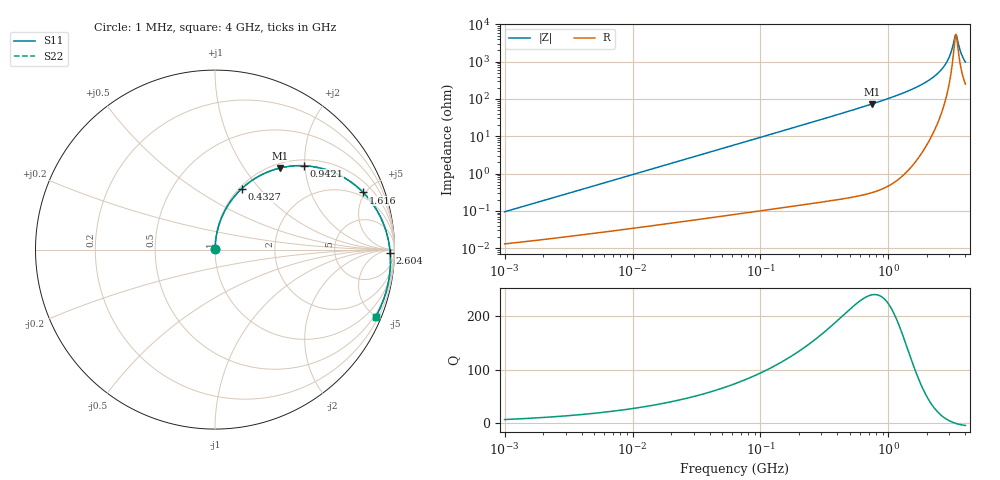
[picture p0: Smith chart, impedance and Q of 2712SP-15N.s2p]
# MHz  S  MA  R  50
!Freq  MagS11  AngS11  MagS21  AngS21  MagS12  AngS12  MagS22  AngS22
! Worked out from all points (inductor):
!   801 points, 1 MHz to 4 GHz, reference 50 ohm
!   read as one part in series: L = 14.9 nH near 1.042 MHz
!   highest Q = 239 at 749.9 MHz (marker M1), where L = 15.7 nH
!   self-resonance near 3.341 GHz
!   S11 on the Smith chart (normalised r, x): 1 MHz: 1.00, +0.00; 432.7 MHz: 1.03, +0.81; 942.1 MHz: 1.13, +1.97; 1.616 GHz: 1.65, +4.84; 2.604 GHz: 48, -41; 4 GHz: 0.38, -4.92
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1  0.0009136 81.8  0.9999 -0.1  0.9999 -0.1  0.0009136 81.8
4.016383  0.003639 86.2  0.9998 -0.2  0.9998 -0.2  0.003639 86.2
15.96482  0.01444 87.4  0.9995 -0.9  0.9995 -0.9  0.01444 87.4
63.45894  0.05729 85.7  0.9976 -3.5  0.9976 -3.5  0.05728 85.7
133.9496  0.1204 82.0  0.9916 -7.4  0.9916 -7.4  0.1203 82.0
252.2445  0.2234 75.8  0.9732 -13.8  0.9732 -13.8  0.2234 75.8
432.659  0.3695 66.4  0.9273 -23.3  0.9273 -23.3  0.3694 66.4
749.8529  0.5814 51.4  0.8112 -38.3  0.8112 -38.3  0.5812 51.4
942.1351  0.6799 43.4  0.7304 -46.3  0.7304 -46.3  0.6797 43.4
1013.11  0.711 40.7  0.7 -49.1  0.7 -49.1  0.7107 40.7
1286.175  0.8074 31.0  0.5852 -58.6  0.5852 -58.6  0.8071 31.0
1615.985  0.885 21.1  0.4568 -68.3  0.4568 -68.3  0.8847 21.1
2138.482  0.9515 8.2  0.2835 -80.2  0.2835 -80.2  0.9512 8.2
2604.497  0.9763 -1.2  0.1586 -87.2  0.1586 -87.2  0.9762 -1.2
2800.706  0.9808 -4.7  0.1134 -88.3  0.1134 -88.3  0.9808 -4.7
2949.842  0.9826 -7.2  0.08179 -87.4  0.08179 -87.4  0.9826 -7.3
3074.848  0.9831 -9.3  0.05734 -84.0  0.05734 -84.0  0.9832 -9.3
3272.36  0.9825 -12.4  0.02486 -59.2  0.02486 -59.2  0.9828 -12.4
3340.977  0.982 -13.5  0.01866 -32.1  0.01866 -32.1  0.9823 -13.5
3446.61  0.9808 -15.1  0.02226 17.7  0.02226 17.7  0.9812 -15.1
3744.916  0.976 -19.4  0.06223 50.2  0.06223 50.2  0.9767 -19.4
4000  0.9706 -22.8  0.09605 52.5  0.09605 52.5  0.9715 -22.8
